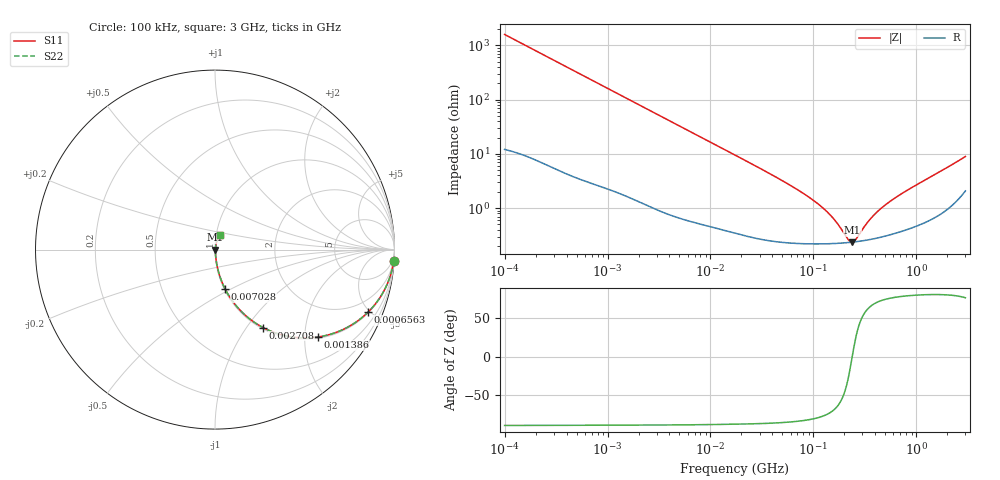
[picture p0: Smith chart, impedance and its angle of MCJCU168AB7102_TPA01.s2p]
! MCJCU168AB7102_TPA01  S-PARAMETER MODEL  ( Standard Model )
! Model Generated by TAIYO YUDEN Corporation (http://www.ty-top.com)
! Version 1.0
! TAIYO YUDEN Control No. 220601
! Copyright(c) 2015 TAIYO YUDEN CO.,LTD. All Rights Reserved.
! Product Description (link to TY-COMPAS)
! https://ds.yuden.co.jp/TYCOMPAS/or/detail?pn=MCJCU168AB7102KTPA01&u=M
! Products Name : Multilayer Ceramic Capacitors
! Characteristics :
!  Capacitance : 1000 [pF] , Rated Voltage : 50 [V] , TCC : X7R
!  Case Size : 1.6 x 0.8 / 0.063 x 0.031 [mm/inch] , Thickness : 0.8 / 0.031 [mm/inch]
!  (Conditions: Temperature = 25 [degC] , DC Bias Voltage = 0 [V])
! External Node Assignments :
!  1  o---| |---o  2
! GND o---------o GND
! Frequency Range : 100kHz  -  3GHz  [ 401 STEP ]
# MHZ S RI R 50
! Freq[MHz].  S11 Real  S11 Imag  S21 Real  S21 Imag  S12 Real  S12 Imag  S22 Real  S22 Imag
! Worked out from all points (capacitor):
!   401 points, 100 kHz to 3 GHz, reference 50 ohm
!   read as one part in series: C = 1 nF near 105.3 kHz
!   lowest |Z| = 236 mohm at 240 MHz (marker M1)
!   series resonance near 238.5 MHz, so ESL is about 440 pH
!   S11 on the Smith chart (normalised r, x): 100 kHz: 1, -32; 656.3 kHz: 1.06, -4.89; 1.386 MHz: 1.04, -2.33; 2.708 MHz: 1.02, -1.20; 7.028 MHz: 1.01, -0.47; 3 GHz: 1.04, +0.17
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0.1  0.9956 -0.0628  0.00444 0.0628  0.00444 0.0628  0.9956 -0.0628
0.246461  0.9752 -0.1506  0.0248 0.1506  0.0248 0.1506  0.9752 -0.1506
0.562235  0.8875 -0.3103  0.1125 0.3103  0.1125 0.3103  0.8875 -0.3103
0.656258  0.8535 -0.3476  0.1465 0.3476  0.1465 0.3476  0.8535 -0.3476
0.941399  0.7417 -0.4309  0.2583 0.4309  0.2583 0.4309  0.7417 -0.4309
1.385689  0.5744 -0.4868  0.4256 0.4868  0.4256 0.4868  0.5744 -0.4868
1.887902  0.4249 -0.4863  0.5751 0.4863  0.5751 0.4863  0.4249 -0.4863
2.708188  0.268 -0.4345  0.732 0.4345  0.732 0.4345  0.268 -0.4345
3.161081  0.2133 -0.401  0.7867 0.401  0.7867 0.401  0.2133 -0.401
4.534557  0.1191 -0.3145  0.8809 0.3145  0.8809 0.3145  0.1191 -0.3145
7.027689  0.0559 -0.2185  0.9441 0.2185  0.9441 0.2185  0.0559 -0.2185
17.7727  0.0118 -0.0912  0.9882 0.0912  0.9882 0.0912  0.0118 -0.0912
51.12795  0.00328 -0.031  0.9967 0.031  0.9967 0.031  0.00328 -0.031
97.38194  0.00239 -0.0142  0.9976 0.0142  0.9976 0.0142  0.00239 -0.0142
143.341  0.00226 -0.00739  0.9977 0.00739  0.9977 0.00739  0.00226 -0.00739
171.6802  0.00226 -0.00465  0.9977 0.00465  0.9977 0.00465  0.00226 -0.00465
216.4987  0.00231 -0.00134  0.9977 0.00134  0.9977 0.00134  0.00231 -0.00134
240.0085  0.00236 8.72e-05  0.9976 -8.72e-05  0.9976 -8.72e-05  0.00236 8.72e-05
259.3015  0.0024 0.00116  0.9976 -0.00116  0.9976 -0.00116  0.0024 0.00116
371.9668  0.00272 0.00629  0.9973 -0.00629  0.9973 -0.00629  0.00272 0.00629
547.5153  0.00334 0.0126  0.9967 -0.0126  0.9967 -0.0126  0.00334 0.0126
3000  0.0274 0.0829  0.9726 -0.0829  0.9726 -0.0829  0.0274 0.0829
